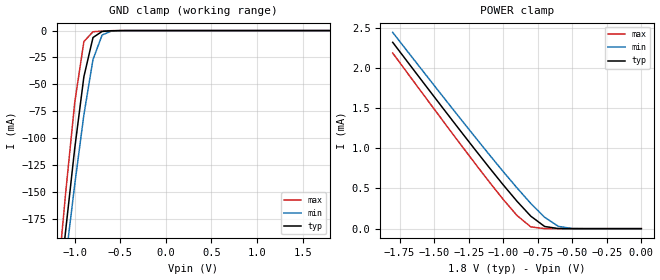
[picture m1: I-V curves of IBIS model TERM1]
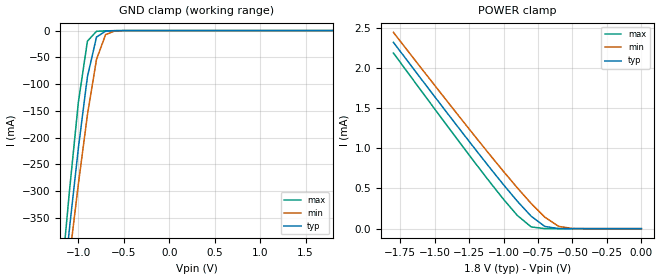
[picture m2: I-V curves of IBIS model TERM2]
|   PERICOM SEMICONDUCTOR CORP
|   IBIS Model of PI4MSD5V9540B
|   Product Family: 4MSD
|   SOIC-8 (W) Package
[IBIS Ver] 3.2
[Comment char] |_char
[File Name] pi4msd5v9540b_w_18v.ibs
[File Rev] 1.0
[Source] File originated at Pericom Semiconductor Corp.
[Date] 09/07/17
[Disclaimer] (C) Copyright PERICOM Semiconductor Corporation
   All rights reserved
  Pericom Semiconductor Corporation hereby grants the user of
  this IBIS model a non-exclusive, nontransferable license to
  use this IBIS model under the following terms.
  This IBIS model is provided on an "AS IS" basis and Pericom
  makes absolutely no warranty with respect to the information
  contained herein. PERICOM DISCLAIMS AND CUSTOMER WAIVES ALL
  WARRANTIES, EXPRESSED OR IMPLIED, INCLUDING WARRANTIES OF
  MERCHANTABILITY OR FITNESS FOR A PARTICULAR PURPOSE. The
  entire risk as to quality and performance is with the customer.
  Accordingly, in no event shall the company be liable for any
  damages, whether in contract or tort, including any lost
  profits or other incidental, consequential, exemplary, or
  punitive damages arising out of the use or application of the
  IBIS model provided in this package. Further, Pericom reserves
  the right to make changes without notice to any product herein
  to improve reliability, function, or design. Pericom does not
  convey any license under patent rights or any other intellectual
  property rights, including those of third parties.
  The user is granted this license only to use the IBIS model
  and is not granted rights to sell, load, rent, lease or license
  the IBIS model in whole or in part, or in modified form to anyone
  other than user. User may modify the IBIS model to suit its specific
  application but rights to derivative works and such modifications
  shall belong to Pericom.
  Pericom is not obligated to provide maintenance or support
  for the licensed IBIS model.
  Contact Pericom at ATTN: APPLICATION ENGINEERING / IBIS MODELS
  2380 Bering Drive, San Jose, CA 95131
[Component] PI4MSD5V9540B
[Manufacturer] Pericom Semiconductor Corp.
[Package]
| variable   typ   min   max
R_pkg   0.05434ohm   0.05079ohm   0.05789ohm
L_pkg   2.52900nH   2.41200nH   2.64600nH
C_pkg   0.17850pF   0.15800pF   0.19900pF
[Pin] signal_name   model_name   R_pin   L_pin   C_pin
1   SCL   TERM2   0.05789   2.64600nH   0.19900pF
2   SDA   TERM2   0.05079   2.41200nH   0.15800pF
3   VCC   POWER   0.05079   2.41200nH   0.15800pF
4   SD0   TERM1   0.05789   2.64600nH   0.19900pF
5   SC0   TERM1   0.05789   2.64600nH   0.19900pF
6   GND   GND   0.05079   2.41200nH   0.15800pF
7   SD1   TERM1   0.05079   2.41200nH   0.15800pF
8   SC1   TERM1   0.05789   2.64600nH   0.19900pF
[Series Switch Groups]
On 1 /
Off 2 /
[Series Pin Mapping]   pin_2   model_name  function_table_group
4   2   SWITCH1   1
5   1   SWITCH1   1
7   2   SWITCH1   2
8   1   SWITCH1   2
|   Model SWITCH1
[Model] SWITCH1
Model_type Series_switch
| variable   typ   min   max
C_comp   7.10pF   7.08pF   7.12pF
[Voltage Range]   1.8000V   1.6200V   1.9800V
[GND Clamp Reference]   0.0000V   0.0000V   0.0000V
[POWER Clamp Reference]   1.8000V   1.6200V   1.9800V
[Temperature Range]   25   85   -40
[On]
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[OFF]
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| Models and submodels in the file (3): SWITCH1 (Series_switch), TERM1 (Terminator), TERM2 (Terminator)
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|   Model TERM1
[Model] TERM1
Model_type Terminator
| variable   typ   min   max
C_comp   2.65pF   2.64pF   2.66pF
[Voltage Range]   1.8000V   1.6200V   1.9800V
[GND Clamp Reference]   0.0000V   0.0000V   0.0000V
[POWER Clamp Reference]   1.8000V   1.6200V   1.9800V
[Temperature Range]   25   85   -40
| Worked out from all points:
|   GND clamp passes 1 mA (typ) near -0.70 V on its own axis
|   POWER clamp passes 1 mA (typ) near -1.21 V on its own axis
[GND Clamp]
| Voltage   I(typ)   I(min)   I(max)
-1.8V     -779.5mA   -743.6mA   -831.9mA
-1.2V     -267.2mA   -286mA     -243.4mA
-1.1V     -186.2mA   -213.2mA   -151.2mA
-1V       -109.4mA   -143.1mA   -66.79mA
-900mV    -42.98mA   -78.43mA   -10.22mA
-800mV    -6.45mA    -26.94mA   -1.105mA
-700mV    -805uA     -4.15mA    -477.3uA
-600mV    -185.9uA   -544.9uA   -115.7uA
1.8V      37.5pA     93.35pA    36.54pA
[POWER Clamp]   |Note: Vtable = Vcc - Voutput
| Voltage   I(typ)   I(min)   I(max)
-1.8V     2.317mA    2.441mA    2.184mA
-1.4V     1.417mA    1.564mA    1.257mA
-1.1V     757.6uA    919.3uA    579.7uA
-1V       544.9uA    710.2uA    363.8uA
-900mV    340.5uA    506.6uA    163.7uA
-800mV    155.1uA    313.2uA    21.83uA
-700mV    27.01uA    141.6uA    235.6nA
-600mV    852.4nA    28.01uA    1.684nA
-500mV    17.64nA    1.596uA    65.36pA
0V        37.5pA     37.78pA    41.21pA
|   Model TERM2
[Model] TERM2
Model_type Terminator
| variable   typ   min   max
C_comp   4.45pF   4.44pF   4.46pF
[Voltage Range]   1.8000V   1.6200V   1.9800V
[GND Clamp Reference]   0.0000V   0.0000V   0.0000V
[POWER Clamp Reference]   1.8000V   1.6200V   1.9800V
[Temperature Range]   25   85   -40
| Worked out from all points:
|   GND clamp passes 1 mA (typ) near -0.70 V on its own axis
|   POWER clamp passes 1 mA (typ) near -1.21 V on its own axis
[GND Clamp]
| Voltage   I(typ)   I(min)   I(max)
-1.8V     -1.564A    -1.492A    -1.669A
-1.2V     -536.3mA   -573.9mA   -488.8mA
-1.1V     -373.8mA   -427.8mA   -304mA
-1V       -219.8mA   -287.2mA   -134.4mA
-900mV    -86.22mA   -157.4mA   -19.74mA
-800mV    -12.06mA   -53.77mA   -1.311mA
-700mV    -1.032mA   -7.522mA   -526.9uA
-600mV    -210.6uA   -734.5uA   -129.9uA
1.8V      68.64pA    148.9pA    67.17pA
[POWER Clamp]   |Note: Vtable = Vcc - Voutput
| Voltage   I(typ)   I(min)   I(max)
-1.8V     2.317mA    2.441mA    2.184mA
-1.4V     1.417mA    1.564mA    1.257mA
-1.1V     757.6uA    919.3uA    579.7uA
-1V       544.9uA    710.2uA    363.8uA
-900mV    340.5uA    506.6uA    163.7uA
-800mV    155.1uA    313.2uA    21.83uA
-700mV    27.01uA    141.6uA    235.7nA
-600mV    852.4nA    28.01uA    1.729nA
-500mV    17.68nA    1.596uA    108.9pA
0V        68.64pA    88.42pA    75.24pA
